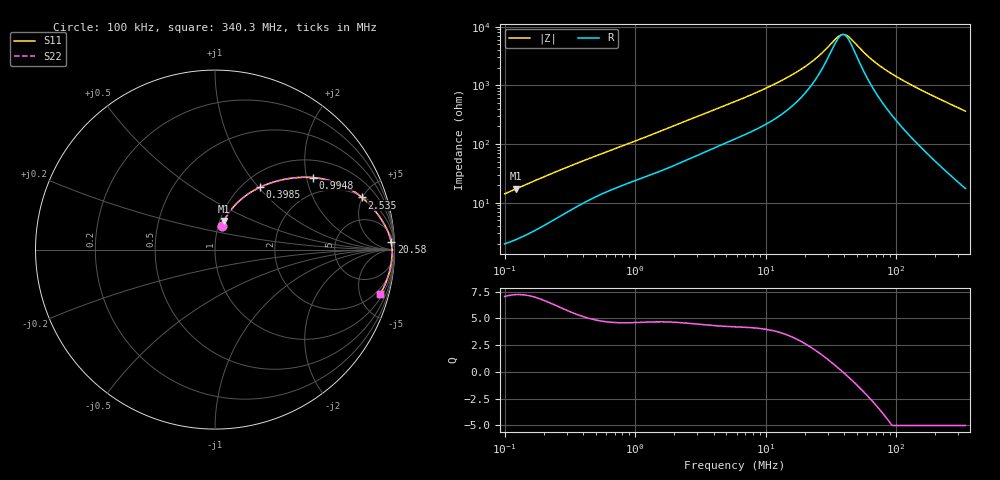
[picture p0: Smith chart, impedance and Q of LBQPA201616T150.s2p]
! LBQPA201616T150  S-PARAMETER MODEL  ( General Type )
! Model Generated by TAIYO YUDEN Corporation (http://www.ty-top.com)
! Version 1.0
! TAIYO YUDEN Control No. 191025NI43SB-FBB
! Copyright(c) 2019 TAIYO YUDEN CO.,LTD. All Rights Reserved.
! Product Description (link to TY-COMPAS)
! https://ds.yuden.co.jp/TYCOMPAS/or/detail?pn=LBQPA201616T150K&u=M
! Products Name : Inductors
! Characteristics :
!  Inductance : 15 uH , SRF(min) : 28 MHz , DC Resistance(max) : 1.56 Ohm
!  Rated Current : Saturation :300 mA , Temp Rise : 255 mA (20 degC)
!  Case Size : 2.0 x 1.6 / 0.079 x 0.063 [mm/inch] , Thickness : 1.6 / 0.063 [mm/inch]
!  (Conditions: Temperature = 25 degC , DC Bias Current/Voltage = 0A / 0V)
! External Node Assignments :
!  1  o---GGG---o  2
! GND o---------o GND
! Frequency Range : 0.1MHz  -  340.31115MHz  [ 402 STEP ]
# MHz S RI R 50
! Freq[MHz].  S11 Real  S11 Imag  S21 Real  S21 Imag  S12 Real  S12 Imag  S22 Real  S22 Imag
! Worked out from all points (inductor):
!   401 points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, 100 kHz to 340.3 MHz, reference 50 ohm
!   read as one part in series: L = 22.2 uH near 104.2 kHz
!   highest Q = 7.23 at 122.5 kHz (marker M1), where L = 22.3 uH
!   self-resonance near 39.12 MHz
!   S11 on the Smith chart (normalised r, x): 100 kHz: 1.04, +0.28; 398.5 kHz: 1.20, +1.02; 994.8 kHz: 1.47, +2.19; 2.535 MHz: 2.09, +4.97; 20.58 MHz: 17, +40; 340.3 MHz: 1.35, -7.28
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0.1  0.0378 0.1326  0.9622 -0.1326  0.9622 -0.1326  0.0378 0.1326
0.122545  0.0498 0.1592  0.9502 -0.1592  0.9502 -0.1592  0.0498 0.1592
0.220983  0.1171 0.2535  0.8829 -0.2535  0.8829 -0.2535  0.1171 0.2535
0.390471  0.244 0.3442  0.756 -0.3442  0.756 -0.3442  0.244 0.3442
0.398491  0.2496 0.3469  0.7504 -0.3469  0.7504 -0.3469  0.2496 0.3469
0.64913  0.3996 0.3939  0.6004 -0.3939  0.6004 -0.3939  0.3996 0.3939
0.994844  0.5467 0.4012  0.4533 -0.4012  0.4533 -0.4012  0.5467 0.4012
1.524679  0.6896 0.3681  0.3104 -0.3681  0.3104 -0.3681  0.6896 0.3681
2.534666  0.8193 0.2903  0.1807 -0.2903  0.1807 -0.2903  0.8193 0.2903
5.953437  0.9312 0.161  0.0688 -0.161  0.0688 -0.161  0.9312 0.161
12.1285  0.9699 0.0839  0.0301 -0.0839  0.0301 -0.0839  0.9699 0.0839
20.57685  0.9818 0.0415  0.0182 -0.0415  0.0182 -0.0415  0.9818 0.0415
22.77862  0.9831 0.0345  0.0169 -0.0345  0.0169 -0.0345  0.9831 0.0345
27.35234  0.9848 0.0224  0.0152 -0.0224  0.0152 -0.0224  0.9848 0.0224
35.62711  0.9863 0.00578  0.0137 -0.00578  0.0137 -0.00578  0.9863 0.00578
37.86776  0.9865 0.00201  0.0135 -0.00201  0.0135 -0.00201  0.9865 0.00201
40.24933  0.9867 -0.00175  0.0133 0.00175  0.0133 0.00175  0.9867 -0.00175
44.5561  0.9868 -0.00807  0.0132 0.00807  0.0132 0.00807  0.9868 -0.00807
65.56488  0.9863 -0.0335  0.0137 0.0335  0.0137 0.0335  0.9863 -0.0335
88.94399  0.9843 -0.0569  0.0157 0.0569  0.0157 0.0569  0.9843 -0.0569
160.3901  0.9732 -0.1184  0.0268 0.1184  0.0268 0.1184  0.9732 -0.1184
340.3111  0.9196 -0.2489  0.0804 0.2489  0.0804 0.2489  0.9196 -0.2489
